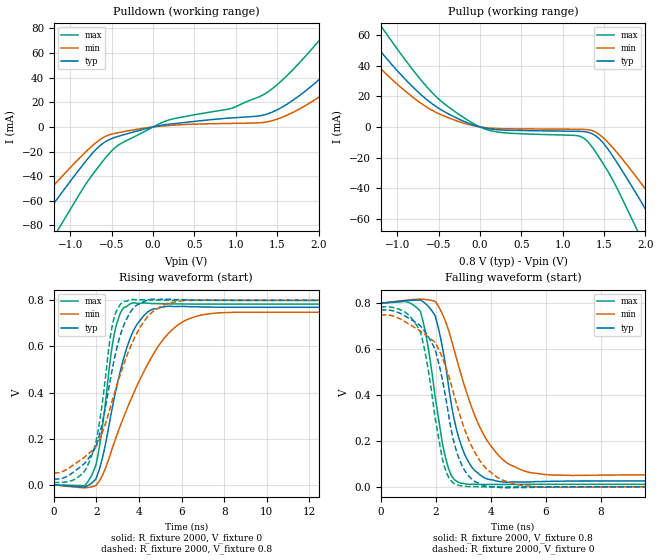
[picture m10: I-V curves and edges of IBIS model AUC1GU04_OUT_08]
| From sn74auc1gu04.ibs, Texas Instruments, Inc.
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[Model]   AUC1GU04_OUT_08
Model_type  Output
Vref =   0
Rref =   2000
Cref =   15p
Vmeas =   0.4
| variable   typ   min   max
C_comp   3.85pF   1.90pF   5.24pF
| C_pullup   3.15pF   1.90pF   4.65pF
| C_pulldown   4.56pF   3.47pF   5.24pF
[Temperature Range]   40   100   -40
| Ambient temperature   25   85   -40
[Voltage range]   0.8   0.8   0.8
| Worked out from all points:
|   slope of the pulldown table from 0 to 0.12 V, typ, clamps not added: 76.8 ohm
|   slope of the pullup table from 0 to 0.12 V, typ, clamps not added: 93.3 ohm
|   rising waveform, R_fixture 2000, V_fixture 0: 20-80 % time 1.13ns typ, 2.17ns min, 660ps max; typ from 0 V to 0.77 V
|   falling waveform, R_fixture 2000, V_fixture 0.8: 20-80 % time 745ps typ, 1.32ns min, 604ps max; typ from 0.8 V to 0.025 V
|   rising waveform, R_fixture 2000, V_fixture 0.8: 20-80 % time 1.08ns typ, 1.69ns min, 727ps max; typ from 0.025 V to 0.8 V
|   falling waveform, R_fixture 2000, V_fixture 0: 20-80 % time 851ps typ, 1.32ns min, 647ps max; typ from 0.77 V to 0 V
[Pulldown]
| AUC1GU04_OUT_08
|   Voltage   I(typ)   I(min)   I(max)
-3.6V     -284.6mA   -233.3mA   -355.2mA
-1.635V   -102.3mA   -80.04mA   -138.1mA
-1.44V    -84.23mA   -65.27mA   -116.3mA
-1.15V    -57.63mA   -43.76mA   -83.72mA
-695mV    -18.59mA   -13.04mA   -35.42mA
-425mV    -7.676mA   -4.712mA   -15mA
170mV     2.015mA    1.069mA    5.198mA
1.32V     9.418mA    3.544mA    25.71mA
2.195V    50.12mA    33.4mA     85.21mA
2.675V    83.38mA    60.83mA    125.3mA
2.97V     105.6mA    80.14mA    150.5mA
7.2V      469.6mA    443.2mA    523mA
[Pullup]
| AUC1GU04_OUT_08
|   Voltage   I(typ)   I(min)   I(max)
-3.6V     236.5mA    214.2mA    262.9mA
-1.68V    82.37mA    66.45mA    104.3mA
-1.44V    65.22mA    51.57mA    84.98mA
-1.21V    49.73mA    38.52mA    66.81mA
-640mV    17.67mA    12.82mA    25.98mA
-80mV     1.281mA    811.3uA    2.224mA
1.255V    -3.057mA   -1.611mA   -7.333mA
1.495V    -10.82mA   -7.315mA   -24.47mA
1.88V     -42.67mA   -31.92mA   -64.88mA
2.15V     -67.12mA   -51.45mA   -95.51mA
2.48V     -97.57mA   -76.17mA   -132.8mA
7.2V      -535.7mA   -447.1mA   -656mA
[Ramp]
| AUC1GU04_OUT_08
| variable   typ   min   max
dV/dt_r   0.47/1.24E-09   0.46/2.19E-09   0.47/7.18E-10
dV/dt_f   0.48/8.22E-10   0.46/1.40E-09   0.48/6.80E-10
R_load = 2000
[Rising Waveform]
| AUC1GU04_OUT_08
R_fixture =   2000
C_fixture =   0
L_fixture =   0
V_fixture =   0
V_fixture_min = 0
V_fixture_max = 0
|   Time   V(typ)   V(min)   V(max)
0s        3.982nV    23.56nV    138.4pV
1.435ns   -9.582mV   -13.2mV    -3.641mV
1.865ns   14.98mV    -6.549mV   59.46mV
2.2ns     87.35mV    26.92mV    199.4mV
2.89ns    399.7mV    197.5mV    676.2mV
3.685ns   657.3mV    384.2mV    788.2mV
4.405ns   749.2mV    522.7mV    787.9mV
5.305ns   773.7mV    648.7mV    784.9mV
7.125ns   771mV      739.5mV    783.7mV
34.99ns   769.9mV    748.6mV    783.8mV
[Falling Waveform]
| AUC1GU04_OUT_08
R_fixture =   2000
C_fixture =   0
L_fixture =   0
V_fixture =   0.8
V_fixture_min = 0.8
V_fixture_max = 0.8
|   Time   V(typ)   V(min)   V(max)
0s        800mV      800mV      800mV
1.435ns   814.3mV    818.1mV    766.3mV
1.7ns     790.3mV    815.5mV    624.5mV
1.965ns   749.2mV    809.4mV    402.1mV
2.43ns    469.9mV    694.9mV    93.71mV
2.92ns    182.6mV    489.9mV    15.56mV
3.405ns   72.42mV    314.6mV    10.67mV
4.205ns   25.31mV    147.3mV    9.912mV
5.955ns   22.94mV    53.31mV    10.42mV
34.99ns   25.46mV    52.25mV    10.6mV
[Rising Waveform]
| AUC1GU04_OUT_08
R_fixture =   2000
C_fixture =   0
L_fixture =   0
V_fixture =   0.8
V_fixture_min = 0.8
V_fixture_max = 0.8
|   Time   V(typ)   V(min)   V(max)
0s        25.46mV    52.25mV    10.6mV
1.07ns    65.29mV    95.74mV    29.07mV
1.725ns   127mV      142.8mV    114mV
2.115ns   208.6mV    190.8mV    254.4mV
2.77ns    513.3mV    373.7mV    700.5mV
3.3ns     695.3mV    526.7mV    795.7mV
3.775ns   770.3mV    634.5mV    803.4mV
4.475ns   803.1mV    736.1mV    801.6mV
6.085ns   802.3mV    798.9mV    800.2mV
34.99ns   800mV      800mV      800mV
[Falling Waveform]
| AUC1GU04_OUT_08
R_fixture =   2000
C_fixture =   0
L_fixture =   0
V_fixture =   0
V_fixture_min = 0
V_fixture_max = 0
|   Time   V(typ)   V(min)   V(max)
0s        770mV      748.6mV    783.8mV
900ps     743.2mV    718.2mV    760.6mV
1.42ns    703.7mV    680.5mV    681.2mV
1.88ns    622mV      639mV      387.3mV
2.335ns   407.4mV    532.5mV    80.79mV
2.61ns    220.9mV    424.6mV    19.73mV
2.89ns    109.9mV    307.9mV    4.508mV
3.8ns     3.576mV    83.64mV    -563.1uV
5.27ns    -3.331mV   3.11mV     -312.3uV
34.99ns   244.2nV    -699nV     41.66nV
